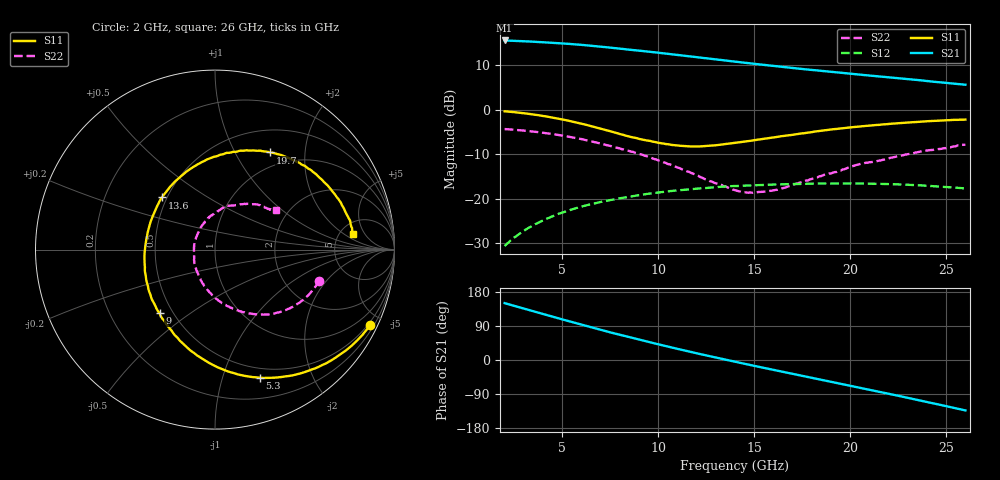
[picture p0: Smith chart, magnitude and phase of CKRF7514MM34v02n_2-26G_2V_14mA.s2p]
! CHUO DENSHI KOGYO Co.,Ltd.
! 22. July 2016
! CKRF7514MM34
! N-channel HJ-FET
! Vds = 2 V Id = 14 mA
# Hz S  MA  R 50
!	f	S11	S21	S12	S22
!	Hz	MAG	ANG	MAG	ANG	MAG	ANG	MAG	ANG
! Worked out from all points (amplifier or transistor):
!   241 points, 2 GHz to 26 GHz, reference 50 ohm
!   highest |S21| = 15.6 dB at 2 GHz (marker M1)
!   |S21| within 3 dB of that: start of sweep to 10.49 GHz
!   unconditionally stable (mu >= 1): 11.9 GHz to 18.82 GHz; 18.93463 GHz to 19.01395 GHz
!   at 6 GHz: K = 0.68, MSG = 18.2 dB, |S12| = -21.8 dB
!   at 14 GHz: K = 1.03, MAG = 13.0 dB, |S12| = -17.2 dB
!   at 26 GHz: K = 0.83, MSG = 11.7 dB, |S12| = -17.7 dB
!   lowest NFmin = 0.37 dB at 10 GHz
!   S11 on the Smith chart (normalised r, x): 2 GHz: 0.39, -4.32; 5.3 GHz: 0.40, -1.33; 9 GHz: 0.42, -0.39; 13.6 GHz: 0.47, +0.33; 19.7 GHz: 0.79, +1.40; 26 GHz: 6.68, +2.84
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2e9  0.961 -25.9  6.01 150.1  0.02929 74.0  0.6068 -16.5
2.9e9  0.92 -37.7  5.9 137.1  0.04203 67.0  0.5856 -23.9
3.7e9  0.8717 -48.6  5.794 125.6  0.05307 60.9  0.5617 -30.6
4.5e9  0.8168 -59.5  5.657 114.3  0.06345 54.9  0.5324 -37.3
5.3e9  0.7554 -70.8  5.51 103.0  0.07337 48.9  0.4994 -44.5
6e9  0.6976 -81.0  5.364 93.3  0.08159 43.6  0.4681 -50.6
6.7e9  0.6382 -91.8  5.195 83.7  0.08884 38.4  0.4323 -56.7
7.5e9  0.5735 -104.6  4.99 73.0  0.09641 32.9  0.3927 -63.9
8.1e9  0.5272 -115.0  4.837 65.2  0.1017 28.7  0.3605 -69.4
9e9  0.4707 -131.1  4.617 53.9  0.1097 23.1  0.3195 -78.3
1e10  0.4255 -151.3  4.377 41.5  0.1174 16.3  0.2698 -89.5
1.08e10  0.4004 -168.2  4.182 31.8  0.123 11.1  0.2334 -98.8
1.17e10  0.3867 172.6  3.97 21.2  0.1281 5.2  0.1953 -111.9
1.26e10  0.3919 154.0  3.768 10.9  0.1326 -0.4  0.1615 -127.5
1.36e10  0.4145 135.5  3.555 -0.3  0.138 -6.8  0.1347 -149.3
1.4e10  0.424 128.5  3.473 -4.6  0.1386 -9.4  0.125 -158.3
1.59e10  0.4851 101.3  3.128 -25.0  0.1442 -21.0  0.1228 151.1
1.8e10  0.5603 77.2  2.804 -46.8  0.1478 -33.7  0.1669 107.7
1.97e10  0.6227 60.4  2.583 -64.7  0.1489 -44.9  0.2147 85.1
2.2e10  0.6925 40.1  2.314 -89.0  0.1459 -60.4  0.2836 61.7
2.4e10  0.743 22.3  2.103 -110.9  0.1398 -75.6  0.3481 45.5
2.6e10  0.7754 6.3  1.911 -133.1  0.1305 -91.4  0.4048 33.0
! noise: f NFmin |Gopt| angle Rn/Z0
1e+10  0.37  0.427  102.4  0.06
1.05e+10  0.39  0.402  111.4  0.06
1.1e+10  0.4  0.37  121.1  0.05
1.15e+10  0.42  0.34  131.6  0.05
1.2e+10  0.45  0.313  144.1  0.04
1.25e+10  0.45  0.294  158  0.04
1.3e+10  0.48  0.281  171.9  0.04
1.35e+10  0.49  0.28  -172.9  0.04
1.4e+10  0.54  0.289  -158.2  0.04
1.5e+10  0.58  0.31  -135.4  0.05
